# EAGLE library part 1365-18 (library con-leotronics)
DUAL ROW STRAIGHT HEADER 1364 SERIES. 1.27mm x 1.27mm. Without Fixing Post. SMT Source: http://www.leotronics.co.uk/Conexcon/Data%20Sheets/sec.%20A/1364ing.pdf
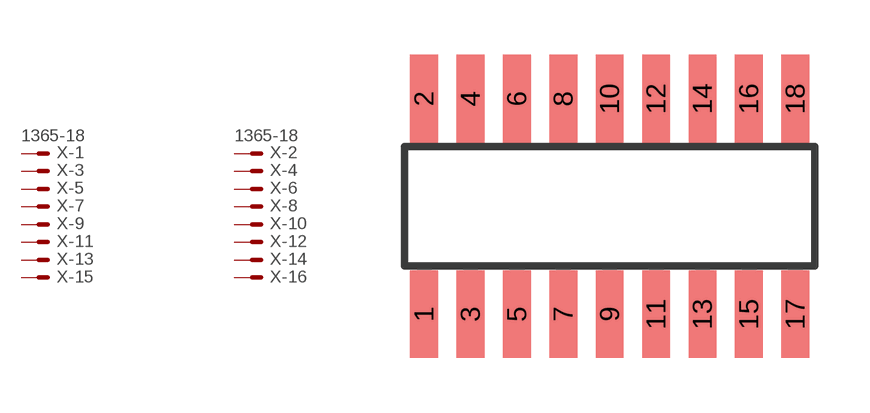
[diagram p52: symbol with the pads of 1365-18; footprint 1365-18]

Designator prefix X; gates -1=MVAL -2=MVAL -3=M -4=M -5=M -6=M -7=M -8=M -9=M -10=M -11=M -12=M -13=M -14=M -15=M -16=M -17=M -18=M

## 1365-18 (OC_FARNELL: unknown; OC_NEWARK: unknown)  [1365-18]
1  -1:S  pas
2  -2:S  pas
3  -3:S  pas
4  -4:S  pas
5  -5:S  pas
6  -6:S  pas
7  -7:S  pas
8  -8:S  pas
9  -9:S  pas
10  -10:S  pas
11  -11:S  pas
12  -12:S  pas
13  -13:S  pas
14  -14:S  pas
15  -15:S  pas
16  -16:S  pas
17  -17:S  pas
18  -18:S  pas

## Footprint 1365-18 (pad centres in mm)
DUAL ROW STRAIGHT HEADER 1364 SERIES. 1.27mm x 1.27mm. Without Fixing Post. SMT Source: http://www.leotronics.co.uk/Conexcon/Data%20Sheets/sec.%20A/1364ing.pdf
smd 0.76 x 2.4: 1 -5.08,-2.95; 2 -5.08,2.95; 3 -3.81,-2.95; 4 -3.81,2.95; 5 -2.54,-2.95; 6 -2.54,2.95; 7 -1.27,-2.95; 8 -1.27,2.95; 9 0,-2.95; 10 0,2.95; 11 1.27,-2.95; 12 1.27,2.95; 13 2.54,-2.95; 14 2.54,2.95; 15 3.81,-2.95; 16 3.81,2.95; 17 5.08,-2.95; 18 5.08,2.95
